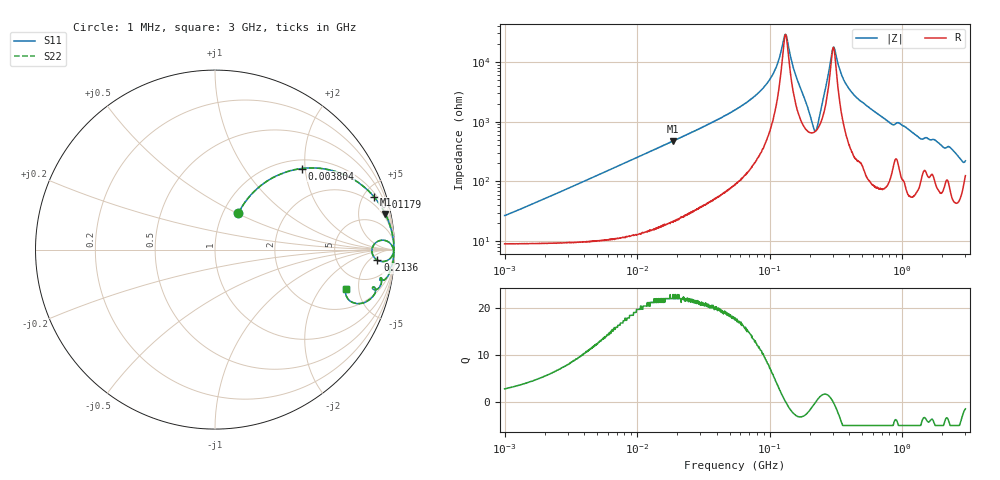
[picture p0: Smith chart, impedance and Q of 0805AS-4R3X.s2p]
!s-Parameter Generated by FASTRON Sdn. Bhd.
!FASTRON P/N : 0805AS-4R3X
!Keysight Technologies: E4991B_MY54100416_A.01.15
!Date: Mon Jun 15 12:59:14 2026
!Version  :Rev01  Mon Jun 15 12:59:14 2026
!Data & Calibration Information:
!Freq  S11  S21  S12  S22
!PortZ  Port1:50+j0  Port2:50+j0
!When reading reference impedance value at option line is always used.
! Remarks : This data is being provided solely for informational purposes.
# Hz S dB R 50
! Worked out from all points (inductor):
!   1601 points, 1 MHz to 3 GHz, reference 50 ohm
!   read as one part in series: L = 4.02 uH near 1.078 MHz
!   highest Q = 22 at 18.68 MHz (marker M1), where L = 4.04 uH
!   self-resonance near 131.5 MHz
!   S11 on the Smith chart (normalised r, x): 1 MHz: 1.18, +0.51; 3.804 MHz: 1.19, +1.92; 11.79 MHz: 1.29, +5.97; 213.6 MHz: 14, -9; 3 GHz: 3.51, -3.66
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1000000  -12.40 57.2  -0.98 -13.1  -0.98 -13.1  -12.40 57.2
1974946  -7.48 55.0  -1.59 -24.6  -1.59 -24.6  -7.48 55.0
3804036  -3.58 43.0  -3.28 -41.2  -3.28 -41.2  -3.58 43.0
1.178658e7  -0.59 18.2  -10.10 -69.0  -10.10 -69.0  -0.59 18.2
1.447069e7  -0.41 15.0  -11.70 -72.3  -11.70 -72.3  -0.41 15.0
1.867766e7  -0.27 11.8  -13.80 -75.7  -13.80 -75.7  -0.27 11.8
5.504702e7  -0.05 3.6  -24.00 -83.2  -24.00 -83.2  -0.05 3.6
9.836149e7  -0.03 1.2  -33.60 -81.5  -33.60 -81.5  -0.03 1.2
1.131553e8  -0.03 0.6  -38.70 -75.2  -38.70 -75.2  -0.03 0.6
1.314834e8  -0.03 0.0  -49.20 -6.2  -49.20 -6.2  -0.03 0.0
1.550909e8  -0.05 -0.8  -36.40 69.0  -36.40 69.0  -0.05 -0.8
2.083556e8  -0.58 -4.1  -20.50 44.9  -20.50 44.9  -0.58 -4.1
2.136344e8  -0.85 -3.7  -19.00 31.7  -19.00 31.7  -0.85 -3.7
2.314421e8  -0.77 3.1  -20.10 -29.8  -20.10 -29.8  -0.77 3.1
2.942768e8  -0.06 0.2  -42.80 -27.3  -42.80 -27.3  -0.06 0.2
3.047674e8  -0.05 -0.1  -44.90 13.6  -44.90 13.6  -0.05 -0.1
3.523638e8  -0.03 -1.0  -35.20 76.8  -35.20 76.8  -0.03 -1.0
4.094372e8  -0.03 -1.8  -30.30 82.2  -30.30 82.2  -0.03 -1.8
7.925923e8  -0.13 -5.7  -20.00 78.8  -20.00 78.8  -0.13 -5.7
2.371269e9  -0.69 -15.2  -11.50 65.8  -11.50 65.8  -0.69 -15.2
2.741597e9  -1.32 -20.5  -8.91 57.0  -8.91 57.0  -1.32 -20.5
3e9  -2.34 -16.5  -9.25 39.1  -9.25 39.1  -2.34 -16.5
